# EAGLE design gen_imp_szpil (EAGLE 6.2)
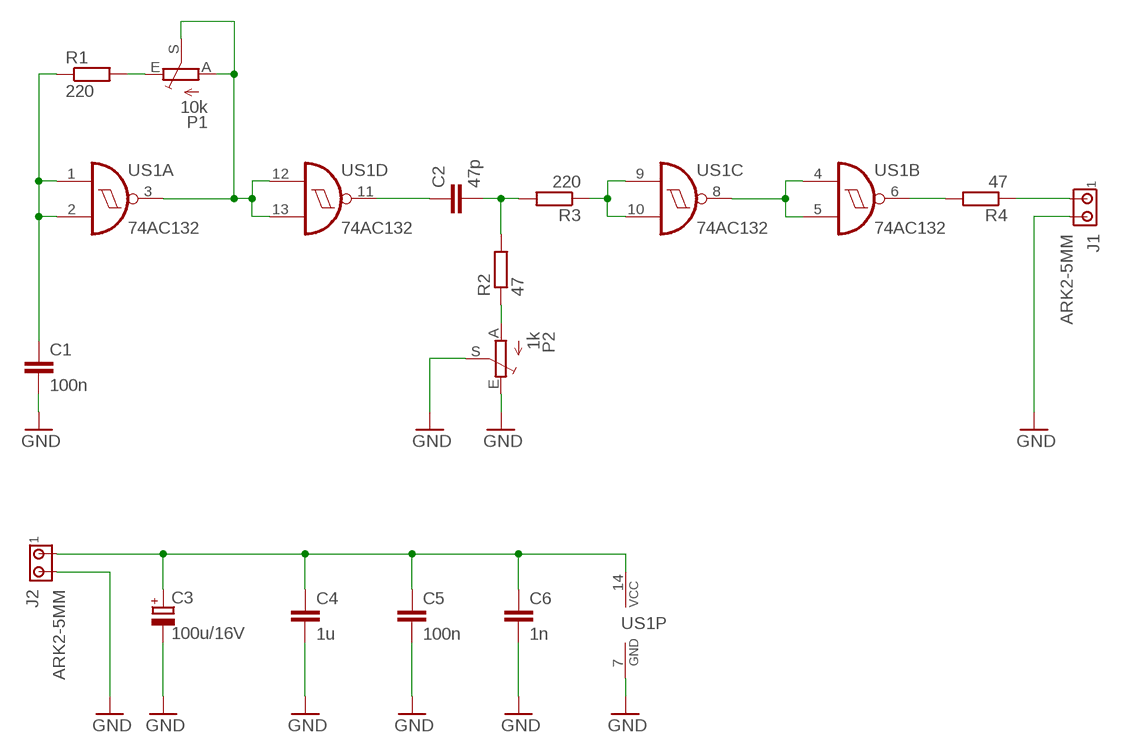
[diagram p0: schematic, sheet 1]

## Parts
C1  100n  C-EUC0805  [C0805]
C2  47p  C-EUC0805  [C0805]
C3  100u/16V  CPOL-EUTT2D5L  [TT2D5L]
C4  1u  C-EUC0805  [C0805]
C5  100n  C-EUC0805  [C0805]
C6  1n  C-EUC0805  [C0805]
J1  ARK2-5MM  [2PIN-5MM]
J2  ARK2-5MM  [2PIN-5MM]
P1  10k  TRIM_EU-B64Y  [B64Y]
P2  1k  TRIM_EU-B64Y  [B64Y]
R1  220  R-EU_M0805  [M0805]
R2  47  R-EU_M0805  [M0805]
R3  220  R-EU_M0805  [M0805]
R4  47  R-EU_M0805  [M0805]
US1  74AC132  74ACT132D  [SO14]

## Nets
GND: C1.2 C3.- C4.2 C5.2 C6.2 J1.P$2 J2.P$2 P2.E P2.S US1.7(P:GND)
N$1: C1.1 R1.1 US1.1(A:I0) US1.2(A:I1)
N$2: P1.E R1.2
N$3: P1.A P1.S US1.3(A:O) US1.12(D:I0) US1.13(D:I1)
N$4: C3.+ C4.1 C5.1 C6.1 J2.P$1 US1.14(P:VCC)
N$6: C2.1 US1.11(D:O)
N$7: C2.2 R2.2 R3.2
N$8: P2.A R2.1
N$9: US1.4(B:I0) US1.5(B:I1) US1.8(C:O)
N$10: R3.1 US1.9(C:I0) US1.10(C:I1)
N$11: J1.P$1 R4.1
N$12: R4.2 US1.6(B:O)

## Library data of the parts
C1 C2 C4-C6 = rcl:C-EU: CAPACITOR, European symbol
C3 = rcl:CPOL-EU: POLARIZED CAPACITOR, European symbol
J1 J2 = zlacza_futrzak:ARK2: ARK 2
P1 P2 = pot:TRIM_EU-: POTENTIOMETER
R1-R4 = rcl:R-EU_: RESISTOR, European symbol
US1 = 74xx-eu:74*132: Quad 2-input NAND schmitt trigger

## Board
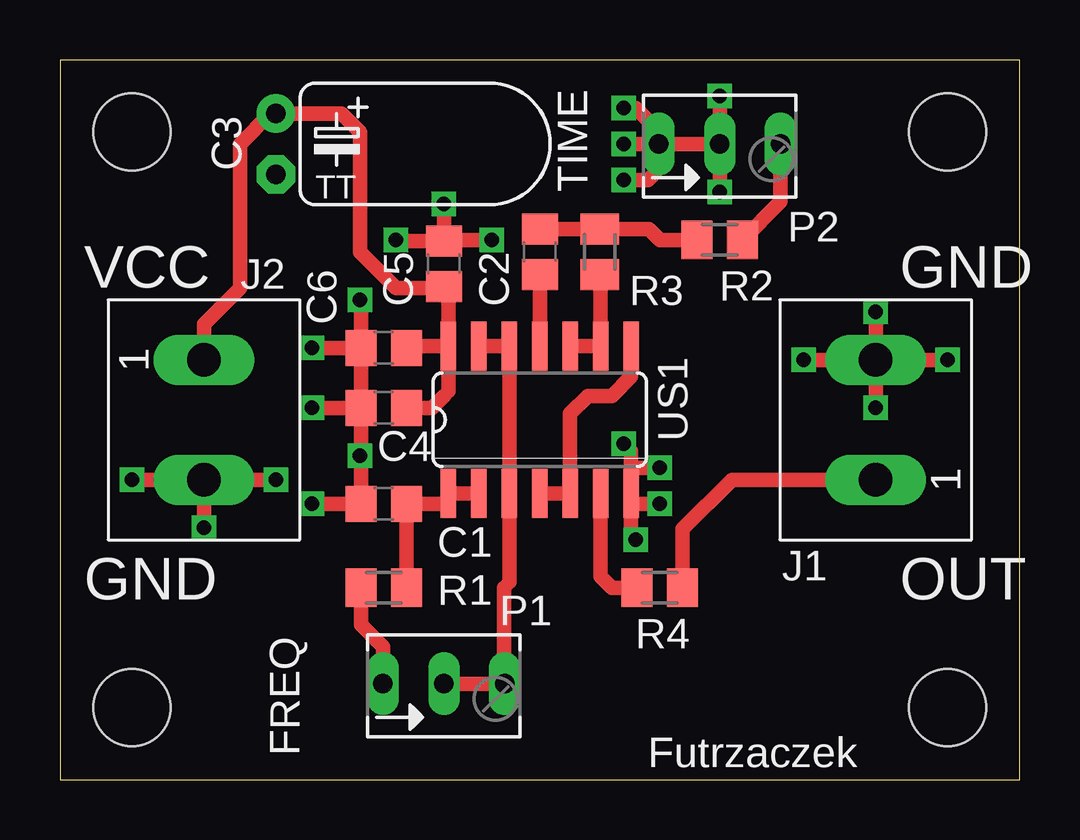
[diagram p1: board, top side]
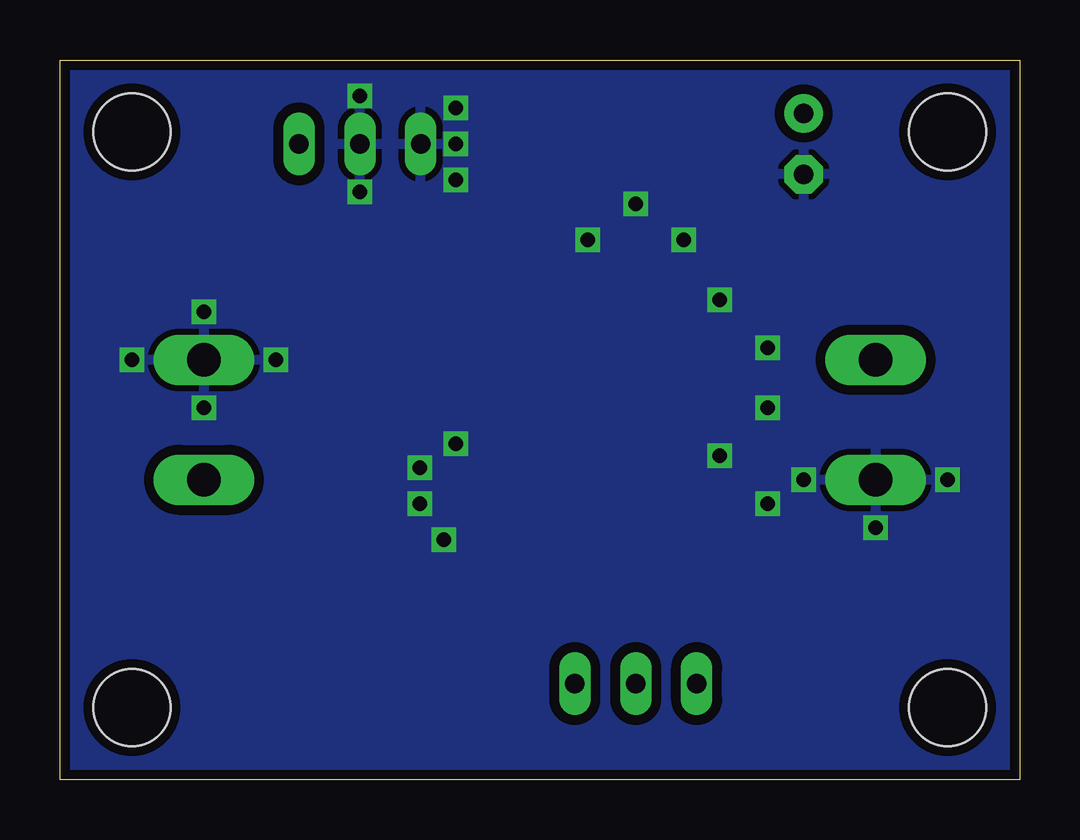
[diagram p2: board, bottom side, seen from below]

Size 40 x 30 mm. Coordinates in mm from the lower left corner, seen from the top.
Outline: 0,0 40,0 40,30 0,30 0,0
Copper layers (1*16): Top 0.035mm / dielectric 1.5mm / Bottom 0.035mm
Design rules: minimum track width 10mil, minimum drill 23mil, track to track 8mil, track to pad 8mil, pad to pad 8mil, via to via 8mil, smd to smd 8mil, copper to edge 15mil, drill to drill 8mil, minimum pad ring 10mil, minimum via ring 8mil, stop-mask expansion 4mil, vias tented up to drill 0mil, thermal gap 10mil
Holes 3.2 mm at 3,3 3,27 37,3 37,27

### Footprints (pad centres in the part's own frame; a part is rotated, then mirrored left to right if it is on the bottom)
C0805 = smd 1.3 x 1.5: 1 -0.95,0; 2 0.95,0
TT2D5L = drill 0.813 pad 1.6: + -1.27,0 | drill 0.813 pad 1.6 octagon: - 1.27,0
2PIN-5MM = drill 1.4 long: P$1 -2.5,0; P$2 2.5,0
B64Y = drill 0.813 long: A 2.54,0; E -2.54,0; S 0,0
M0805 = smd 1.3 x 1.6: 1 -0.95,0; 2 0.95,0
SO14 = smd 0.66 x 2.032: 1 -3.81,-3.073; 2 -2.54,-3.073; 3 -1.27,-3.073; 4 0,-3.073; 5 1.27,-3.073; 6 2.54,-3.073; 7 3.81,-3.073; 8 3.81,3.073; 9 2.54,3.073; 10 1.27,3.073; 11 0,3.073; 12 -1.27,3.073; 13 -2.54,3.073; 14 -3.81,3.073

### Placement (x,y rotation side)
C1  13.5,11.5 180 top
C2  20,22 90 top
C3  9,26.5 270 top
C4  13.5,15.5 180 top
C5  16,21.5 90 top
C6  13.5,18 180 top
J1  34,15 90 top
J2  6,15 270 top
P1  16,4 0 top
P2  27.5,26.5 0 top
R1  13.5,8 180 top
R2  27.5,22.5 180 top
R3  22.5,22 90 top
R4  25,8 180 top
US1  20,15 0 top

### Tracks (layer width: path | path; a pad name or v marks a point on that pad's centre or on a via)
GND  (via drill 0.6)
  Top 0.61: v10.5,15.5 12.5,15.5 | C6.2 v10.5,18 | C6.2 12.55,19.95 v12.5,20 | C6.2 C4.2 12.55,13.55 v12.5,13.5 12.55,13.45 C1.2 v10.5,11.5 | C5.2 14.05,22.45 v14,22.5 | v16,24 16,22.5 v18,22.5 | P2.S P2.E | P2.E v23.5,26.5 | v23.5,25 24.5,25 24.96,25.46 P2.E | v23.5,28 24,28 24.96,27.04 P2.E | v27.5,28.5 P2.S | v27.5,24.5 P2.S | v3,12.5 J2.P$2 | v6,10.5 J2.P$2 | v9,12.5 J2.P$2 | v31,17.5 J1.P$2 | v34,15.5 J1.P$2 | v37,17.5 J1.P$2 | v34,19.5 J1.P$2 | US1.7 23.81,10.19 v24,10 | v25,11.5 24,11.5 23.81,11.69 US1.7 | v23.5,14 23.81,13.69 23.81,13 | 23.81,13 US1.7 | v25,13 23.81,13
  pour Bottom (isolate 0.406): 0,0 40,0 40,30 0,30
N$1
  Top 0.61: US1.2 US1.1 16.19,11.69 16,11.5 C1.1 R1.1
N$2
  Top 0.61: P1.E 13.46,5.54 13,6 12.55,6.45 R1.2
N$3
  Top 0.61: P1.S P1.A 18.5,4.04 18.5,8 18.73,8.23 US1.3 US1.12 US1.13
N$4
  Top 0.61: US1.14 16.19,20.36 C5.1 15.95,20.5 14,20.5 12.5,22 12.5,27 11.73,27.77 8.77,27.77 | US1.14 14.52,18.07 C6.1 | C4.1 15.5,15.5 16,16 16.19,16.19 US1.14 | J2.P$1 6,19 7.5,20.5 7.5,26.5 8.77,27.77 | 8.77,27.77 C3.+ 8.77,27.77
N$6
  Top 0.61: US1.11 C2.1
N$7
  Top 0.61: C2.2 R3.2 24.55,22.95 25,22.5 R2.2
N$8
  Top 0.61: P2.A 30.04,24.09 R2.1
N$9
  Top 0.61: US1.8 23.81,16.81 23,16 22,16 21.27,15.27 US1.5 US1.4
N$10
  Top 0.61: US1.10 US1.9 22.54,21.01 R3.1
N$11
  Top 0.61: R4.1 25.95,10.45 28,12.5 J1.P$1
N$12
  Top 0.61: US1.6 22.54,8.46 23,8 R4.2

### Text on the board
tPlace: TIME | VCC | GND | GND | OUT | FREQ | Futrzaczek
